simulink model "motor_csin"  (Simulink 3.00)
settings: Solver=ode45  StartTime=0.0  StopTime=2.5  RelTol=1e-6  AbsTol=1e-6
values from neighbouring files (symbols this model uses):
  A = [-Ra Xq ; -Xdp -Ra]    [Gsinc.m]    (also in Cinic.m = -Xs*(Xm+Xr)-Xr*Xm; ptaylor.m = 0; Tdqf.m = [sin(u(3)) cos(u(3)); - cos(u(3)) sin(u(3))]; Tfdq.m = [sin(u(3)) cos(u(3)); - cos(u(3)) sin(u(3))])
  Ac = real(z(1,1))    [ptaylor.m]    (also in workspace_ctes.m = 0.0095)
  As = real(z(1,1))    [ptaylor.m]    (also in workspace_ctes.m = 0.035)
  B = [0 u(3)]'    [Gsinc.m]    (also in Cinic.m = Rs*(Xm+Xr); ptaylor.m = 0; workspace_ctes.m = 0)
  Bc = imag(z(1,1))    [ptaylor.m]    (also in workspace_ctes.m = 0.1279)
  Bs = imag(z(1,1))    [ptaylor.m]    (also in workspace_ctes.m = 0.2438)
  C = Pm*A^2+Pm*B^2-Rs*(Xm+Xr)^2    [Cinic.m]    (also in ptaylor.m = 0; workspace_ctes.m = 0)
  Cc = real(z(2,1))    [ptaylor.m]    (also in workspace_ctes.m = -0.3544)
  Cs = real(z(2,1))    [ptaylor.m]    (also in workspace_ctes.m = -0.678)
  D = 2*Pm*Rs*Rr*A+2*Pm*(Xs*Rr+Rr*Xm)*B-Rr*Xm^2    [Cinic.m]    (also in ptaylor.m = 0; workspace_ctes.m = 0)
  Dc = imag(z(2,1))    [ptaylor.m]    (also in workspace_ctes.m = 0.0093)
  Ds = imag(z(2,1))    [ptaylor.m]    (also in workspace_ctes.m = 0.0644)
  Imv = Imv'    [ptaylor.m]    (also in workspace_ctes.m = [-0.0879 -1.7628 -0.2794 1.4912])
  Imvc = Imvc'    [ptaylor.m]    (also in workspace_ctes.m = [-0.0175 -0.6693 -0.2556 1.8032])
  Imvs = Imvs'    [ptaylor.m]    (also in workspace_ctes.m = [-0.1217 -1.2805 -0.3651 0.9022])
  U3v = U3v'    [ptaylor.m]    (also in workspace_ctes.m = [0.6354 -0.0622 0.4667 -0.0233])
  U3vc = U3vc'    [ptaylor.m]    (also in workspace_ctes.m = [0.2415 -0.0179 0.3544 -0.0093])
  U3vs = U3vs'    [ptaylor.m]    (also in workspace_ctes.m = [0.4605 -0.0661 0.6780 -0.0644])

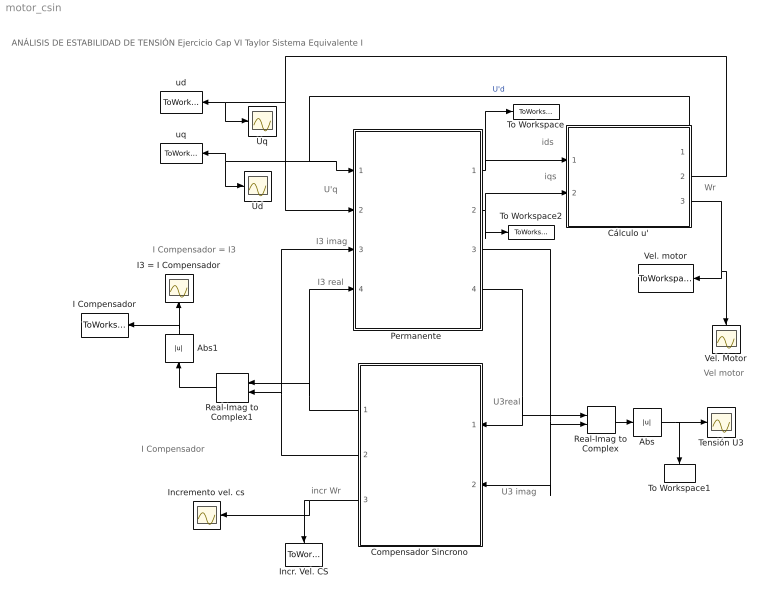
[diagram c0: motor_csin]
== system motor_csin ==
  note: incr Wr
  note: I3 real
  note: I3 imag
  note: U3real
  note: U3 imag
  note: U'q
  note: ids
  note: iqs
  note: Wr
  note: Vel motor
  note: I Compensador
  note: I Compensador = I3
  note: ANÁLISIS DE ESTABILIDAD DE TENSIÓN Ejercicio Cap VI Taylor Sistema Equivalente I
  Abs : Abs
  Abs1 : Abs  Orientation=up
  Compensador Sincrono : Subsystem  Orientation=left  mask{Xd=5.544, Xq=3.26, Xdp=1.14, Ra=0, H=0.5375, Xt=0.34, Emin=-9, Emax=12.43, Tdp=9.564, K=100}
      mask prompts: Xd "Reactancia Síncrona  de Eje d ,  Xd  (p.u.)"; Xq "Reactancia Síncrona  de Eje q,  Xq  (p.u.)"; Xdp "Reactancia Subtransitoria de eje d,  X'd  (p.u.)"; Ra "Resistencia de Estator,  Ra  (p.u.)"; H "Constante de Inercia H (s)"; Xt "Reactancia del transformador,  Xt  (p.u.)"; Emin "Limite Inferior Regulador de Tensión"; Emax "Límite Superior Regulador"; Tdp "Constante de Tiempo del Rotor (s)"; K "Ganancia del Regulador"
  Cálculo u' : Subsystem  mask(Modelo del rotor  del motor){Um=1, Pm=0.6, Am=1, Bm=0, Cm=0, Dm=0, Hm=0.7, Xm=3.2, Xr=0.18, Rr=0.018, Xs=0.1, Rs=0.031}
      mask prompts: Um "Tensión de alimentación (p.u)"; Pm "Potencia en el eje (p.u.)"; Am "Parámetro A modelo de Tcarga"; Bm "Parámetro B modelo de Tcarga"; Cm "Parámetro C modelo de Tcarga"; Dm "Parámetro D modelo de Tcarga"; Hm "Inercia,  H (s)"; Xm "Reactancia de Magnetización,  Xm (p.u.)"; Xr "Reactancia Rotor,  Xr  (p.u.)"; Rr "Resistencia del Rotor,  Rr  (p.u.)"; Xs "Reactancia del estator,  Xs  (p.u.)"; Rs "Resistencia del estator,  Rs  (p.u.)"
  I Compensador : ToWorkspace  VariableName=ICS  SampleTime=-1  SaveFormat=Matrix
  I3 = I Compensador : Scope
  Incr. Vel. CS : ToWorkspace  VariableName=Wmcs  SampleTime=-1  SaveFormat=Matrix
  Incremento vel. cs : Scope
  "Permanente " : Subsystem
  Real-Imag to Complex : RealImagToComplex  Input=RealAndImag  ConstantPart=0
  Real-Imag to Complex1 : RealImagToComplex  Orientation=left  Input=RealAndImag  ConstantPart=0
  Tensión U3 : Scope
  To Workspace : ToWorkspace  VariableName=ids  SampleTime=0  SaveFormat=Matrix
  To Workspace1 : ToWorkspace  VariableName=U3  SampleTime=-1  SaveFormat=Matrix
  To Workspace2 : ToWorkspace  VariableName=iqs  SampleTime=0  SaveFormat=Matrix
  Ud : Scope
  Uq : Scope
  Vel. Motor : Scope
  Vel. motor : ToWorkspace  VariableName=wr  SampleTime=-1  SaveFormat=Matrix
  ud : ToWorkspace  VariableName=uq  SampleTime=-1  SaveFormat=Matrix
  uq : ToWorkspace  VariableName=ud  SampleTime=-1  SaveFormat=Matrix
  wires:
  Compensador Sincrono/2(I3imag) -> "Permanente "/3(I3imag), Real-Imag to Complex1/2
  Compensador Sincrono/1(I3real) -> "Permanente "/4(I3real), Real-Imag to Complex1/1
  "Permanente "/4(U3real) -> Compensador Sincrono/1(U3real), Real-Imag to Complex/1
  "Permanente "/3(U3 imag) -> Compensador Sincrono/2(U3imag), Real-Imag to Complex/2
  Real-Imag to Complex/1 -> Abs/1
  Abs/1 -> Tensión U3/1, To Workspace1/1
  Cálculo u'/2(u'q) -> "Permanente "/2(u'q), ud/1, Uq/1
  Cálculo u'/1(u'd) -> "Permanente "/1(u'd), uq/1, Ud/1  "U'd"
  Compensador Sincrono/3(Inc Wr) -> Incr. Vel. CS/1, Incremento vel. cs/1
  Cálculo u'/3(wr) -> Vel. motor/1, Vel. Motor/1
  "Permanente "/1(ids) -> Cálculo u'/1(ids), To Workspace/1
  "Permanente "/2(iqs) -> Cálculo u'/2(iqs), To Workspace2/1
  Real-Imag to Complex1/1 -> Abs1/1
  Abs1/1 -> I3 = I Compensador/1, I Compensador/1

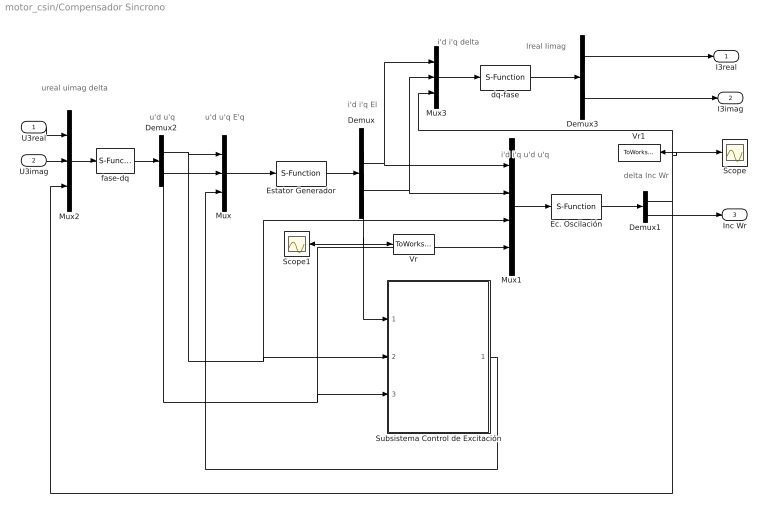
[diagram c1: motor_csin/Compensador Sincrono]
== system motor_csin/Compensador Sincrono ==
  note: u'd u'q E'q
  note: i'd i'q El
  note: i'd i'q u'd u'q
  note: delta Inc Wr
  note: ureal uimag delta
  note: u'd u'q
  note: i'd i'q delta
  note: Ireal Iimag
  U3real : Inport  Port=1  PortWidth=-1  SampleTime=-1  DataType=auto
  U3imag : Inport  Port=2  PortWidth=-1  SampleTime=-1  DataType=auto
  Demux : Demux  Outputs=3
  Demux1 : Demux  Outputs=2
  Demux2 : Demux  Outputs=2
  Demux3 : Demux  Outputs=2
  Ec. Oscilación : S-Function  FunctionName=geosc  Parameters=H  PortCounts=[]  SFunctionModules=''
  Estator Generador : S-Function  FunctionName=gsinc  Parameters=Ra, Xd, Xq, Xdp, Xt  PortCounts=[]  SFunctionModules=''
  Mux : Mux  Inputs=3
  Mux1 : Mux  Inputs=4
  Mux2 : Mux  Inputs=3
  Mux3 : Mux  Inputs=3
  Scope : Scope
  Scope1 : Scope
  Subsistema Control de Excitación : Subsystem  mask{Tdp=Tdp, Emax=Emax, Emin=Emin, K=K}
      mask prompts: Tdp "Cte. Tiempo Rotor"; K "Ganancia Regulador"
  Vr : ToWorkspace  VariableName=El  SampleTime=-1  SaveFormat=Matrix
  Vr1 : ToWorkspace  VariableName=delta  SampleTime=-1  SaveFormat=Matrix
  dq-fase : S-Function  FunctionName=Tdqf  PortCounts=[]  SFunctionModules=''
  fase-dq : S-Function  FunctionName=Tfdq  PortCounts=[]  SFunctionModules=''
  I3real : Outport  Port=1
  I3imag : Outport  Port=2
  Inc Wr : Outport  Port=3
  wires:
  Mux3/1 -> dq-fase/1
  dq-fase/1 -> Demux3/1
  Demux3/1 -> I3real/1
  Demux3/2 -> I3imag/1
  Mux1/1 -> Ec. Oscilación/1
  Demux/1 -> Mux1/1, Mux3/1
  Demux/2 -> Mux1/2, Mux3/2
  Estator Generador/1 -> Demux/1
  Mux2/1 -> fase-dq/1
  U3real/1 -> Mux2/1
  U3imag/1 -> Mux2/2
  fase-dq/1 -> Demux2/1
  Demux2/1 -> Mux/1, Subsistema Control de Excitación/2(u'd), Mux1/3
  Demux2/2 -> Mux/2, Subsistema Control de Excitación/3(u'q), Mux1/4
  Mux/1 -> Estator Generador/1
  Subsistema Control de Excitación/1(E'q) -> Mux/3
  Ec. Oscilación/1 -> Demux1/1
  Demux1/2 -> Inc Wr/1
  Demux1/1 -> Mux2/3, Mux3/3, Scope/1, Vr1/1
  Demux/3 -> Subsistema Control de Excitación/1(E l), Scope1/1, Vr/1

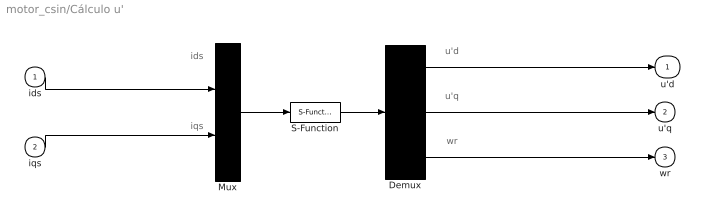
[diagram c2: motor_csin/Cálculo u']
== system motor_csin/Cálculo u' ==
  note: wr
  note: u'q
  note: u'd
  note: iqs
  note: ids
  ids : Inport  Port=1  PortWidth=-1  SampleTime=-1  DataType=auto
  iqs : Inport  Port=2  PortWidth=-1  SampleTime=-1  DataType=auto
  Demux : Demux  Outputs=3
  Mux : Mux  Inputs=2
  S-Function : S-Function  FunctionName=rotorind  Parameters=Rs, Xs, Rr, Xr, Xm, Hm, Am, Bm, Cm, Dm, Pm, Um  PortCounts=[]  SFunctionModules=''
  u'd : Outport  Port=1
  u'q : Outport  Port=2
  wr : Outport  Port=3
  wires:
  ids/1 -> Mux/1
  iqs/1 -> Mux/2
  S-Function/1 -> Demux/1
  Mux/1 -> S-Function/1
  Demux/1 -> u'd/1
  Demux/2 -> u'q/1
  Demux/3 -> wr/1

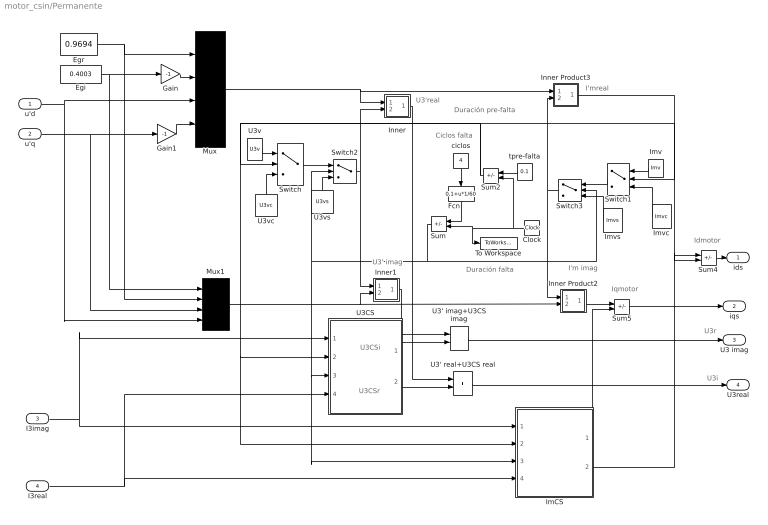
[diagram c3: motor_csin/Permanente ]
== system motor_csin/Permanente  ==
  note: U3'real
  note: U3' imag
  note: I'mreal
  note: I'm imag
  note: Idmotor
  note: U3CSi
  note: U3CSr
  note: Iqmotor
  note: U3r
  note: U3i
  note: Ciclos falta
  note: Duración pre-falta
  note: Duración falta
  u'd : Inport  Port=1  PortWidth=-1  SampleTime=-1  DataType=auto
  u'q : Inport  Port=2  PortWidth=-1  SampleTime=-1  DataType=auto
  I3imag : Inport  Port=3  PortWidth=-1  SampleTime=-1  DataType=auto
  I3real : Inport  Port=4  PortWidth=-1  SampleTime=-1  DataType=auto
  Clock : Clock
  Egi : Constant  Value=0.4003
  Egr : Constant  Value=0.9694
  Fcn : Fcn  Orientation=down  Expr=0.1+u*1/60
  Gain : Gain  Gain=-1  SaturateOnIntegerOverflow=on
  Gain1 : Gain  Gain=-1  SaturateOnIntegerOverflow=on
  ImCS : Subsystem
  Imv : Constant  Orientation=left  Value=Imv
  Imvc : Constant  Orientation=left  Value=Imvc
  Imvs : Constant  Orientation=left  Value=Imvs
  Inner : Subsystem
  Inner Product2 : Subsystem
  Inner Product3 : Subsystem
  Inner1 : Subsystem
  Mux : Mux  Inputs=4
  Mux1 : Mux  Inputs=4
  Sum : Sum  Orientation=left  Inputs=+-  SaturateOnIntegerOverflow=on
  Sum2 : Sum  Orientation=left  Inputs=+-  SaturateOnIntegerOverflow=on
  Sum4 : Sum  Inputs=+-  SaturateOnIntegerOverflow=on
  Sum5 : Sum  Inputs=+-  SaturateOnIntegerOverflow=on
  Switch : Switch  Threshold=0
  Switch1 : Switch  Orientation=left  Threshold=0
  Switch2 : Switch  Threshold=0
  Switch3 : Switch  Orientation=left  Threshold=0
  To Workspace : ToWorkspace  VariableName=t  SampleTime=0  SaveFormat=Matrix
  U3' imag+U3CS imag : Sum  Inputs=++  SaturateOnIntegerOverflow=on
  U3' real+U3CS real : Sum  Inputs=++  SaturateOnIntegerOverflow=on
  U3CS : Subsystem
  U3v : Constant  Value=U3v
  U3vc : Constant  Orientation=up  Value=U3vc
  U3vs : Constant  Orientation=up  Value=U3vs
  ciclos : Constant  Orientation=down  Value=4
  tpre-falta : Constant  Orientation=left  Value=0.1
  ids : Outport  Port=1
  iqs : Outport  Port=2
  U3 imag : Outport  Port=3
  U3real : Outport  Port=4
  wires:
  U3vc/1 -> Switch/3
  U3v/1 -> Switch/1
  Switch/1 -> Switch2/1
  U3vs/1 -> Switch2/3
  Sum/1 -> Switch3/2, Switch2/2, ImCS/3(T falta), U3CS/3(T falta)
  Imvc/1 -> Switch1/3
  Imv/1 -> Switch1/1
  Fcn/1 -> Sum/1
  tpre-falta/1 -> Sum2/1
  Sum2/1 -> Switch1/2, Switch/2, ImCS/2(T pre-falta), U3CS/2(T Pre-falta)
  Switch1/1 -> Switch3/1
  Imvs/1 -> Switch3/3
  ciclos/1 -> Fcn/1
  Inner Product3/1(out_1) -> Sum4/1
  Egr/1 -> Mux/1, Mux1/2
  Mux1/1 -> Inner Product2/2(in_2), Inner1/2(in_2)
  Inner/1(out_1) -> U3' real+U3CS real/1
  U3CS/2(U3CS real) -> U3' real+U3CS real/2
  U3CS/1(U3CS imag.) -> U3' imag+U3CS imag/2
  Inner1/1(out_1) -> U3' imag+U3CS imag/1
  Inner Product2/1(out_1) -> Sum5/1
  I3real/1 -> ImCS/4(I3 real), U3CS/4(I3 real)
  I3imag/1 -> ImCS/1(I3 imag.), U3CS/1(I3 imag.)
  Sum4/1 -> ids/1
  Sum5/1 -> iqs/1
  U3' imag+U3CS imag/1 -> U3 imag/1
  U3' real+U3CS real/1 -> U3real/1
  Gain1/1 -> Mux/4
  u'q/1 -> Gain1/1, Mux1/3
  u'd/1 -> Mux/3, Mux1/4
  Gain/1 -> Mux/2
  Egi/1 -> Gain/1, Mux1/1
  Switch3/1 -> Inner Product2/1(in_1), Inner Product3/2(in_2)
  Switch2/1 -> Inner1/1(in_1), Inner/2(in_2)
  Mux/1 -> Inner Product3/1(in_1), Inner/1(in_1)
  Clock/1 -> Sum/2, To Workspace/1, Sum2/2
  ImCS/2(ImCS real) -> Sum4/2
  ImCS/1(ImCS imag) -> Sum5/2

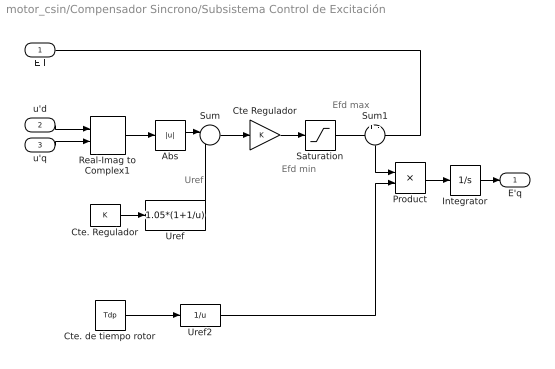
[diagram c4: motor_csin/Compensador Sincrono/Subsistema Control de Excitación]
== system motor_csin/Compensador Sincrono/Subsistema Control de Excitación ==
  note: Uref
  note: Efd max
  note: Efd min
  E l : Inport  Port=1  PortWidth=-1  SampleTime=-1  DataType=auto
  u'd : Inport  Port=2  PortWidth=-1  SampleTime=-1  DataType=auto
  u'q : Inport  Port=3  PortWidth=-1  SampleTime=-1  DataType=auto
  Abs : Abs
  Cte Regulador : Gain  Gain=K  SaturateOnIntegerOverflow=on
  Cte. Regulador : Constant  Value=K
  Cte. de tiempo rotor : Constant  Value=Tdp
  Integrator : Integrator  ExternalReset=none  InitialConditionSource=internal  InitialCondition=1.05  LimitOutput=off  UpperSaturationLimit=inf  LowerSaturationLimit=-inf  ShowSaturationPort=off  ShowStatePort=off  AbsoluteTolerance=auto
  Product : Product  Inputs=2  SaturateOnIntegerOverflow=on
  Real-Imag to Complex1 : RealImagToComplex  Input=RealAndImag  ConstantPart=0
  Saturation : Saturate  UpperLimit=Emax  LowerLimit=Emin
  Sum : Sum  Inputs=|-+  SaturateOnIntegerOverflow=on
  Sum1 : Sum  Orientation=down  Inputs=+-  SaturateOnIntegerOverflow=on
  Uref : Fcn  Expr=1.05*(1+1/u)
  Uref2 : Fcn  Expr=1/u
  E'q : Outport  Port=1
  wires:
  Sum/1 -> Cte Regulador/1
  Cte Regulador/1 -> Saturation/1
  Abs/1 -> Sum/1
  Cte. Regulador/1 -> Uref/1
  Uref/1 -> Sum/2
  Saturation/1 -> Sum1/1
  E l/1 -> Sum1/2
  Product/1 -> Integrator/1
  Integrator/1 -> E'q/1
  Sum1/1 -> Product/1
  Cte. de tiempo rotor/1 -> Uref2/1
  Uref2/1 -> Product/2
  Real-Imag to Complex1/1 -> Abs/1
  u'd/1 -> Real-Imag to Complex1/1
  u'q/1 -> Real-Imag to Complex1/2

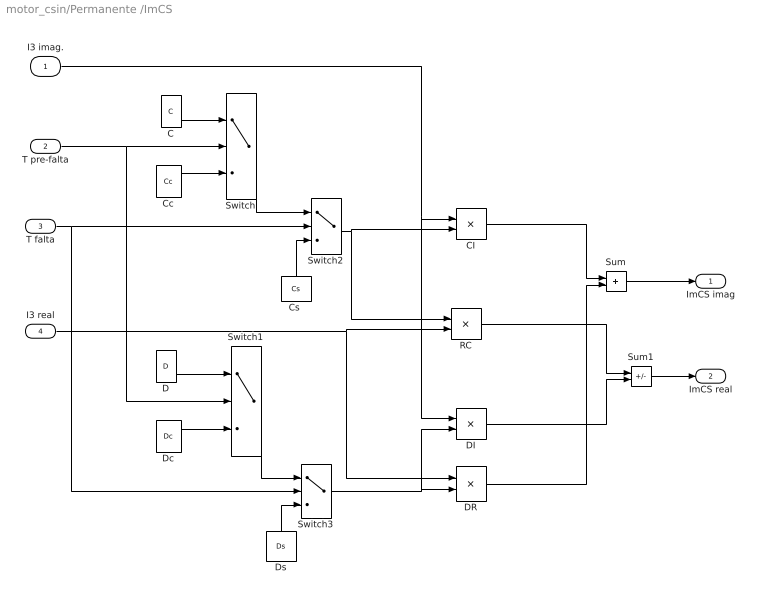
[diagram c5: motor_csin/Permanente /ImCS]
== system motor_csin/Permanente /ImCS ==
  I3 imag. : Inport  Port=1  PortWidth=-1  SampleTime=-1  DataType=auto
  T pre-falta : Inport  Port=2  PortWidth=-1  SampleTime=-1  DataType=auto
  T falta : Inport  Port=3  PortWidth=-1  SampleTime=-1  DataType=auto
  I3 real : Inport  Port=4  PortWidth=-1  SampleTime=-1  DataType=auto
  C : Constant  Value=C
  CI : Product  Inputs=2  SaturateOnIntegerOverflow=on
  Cc : Constant  Value=Cc
  "Cs " : Constant  Orientation=up  Value=Cs
  D : Constant  Value=D
  DI : Product  Inputs=2  SaturateOnIntegerOverflow=on
  DR : Product  Inputs=2  SaturateOnIntegerOverflow=on
  Dc : Constant  Value=Dc
  Ds : Constant  Orientation=up  Value=Ds
  RC : Product  Inputs=2  SaturateOnIntegerOverflow=on
  Sum : Sum  Inputs=++  SaturateOnIntegerOverflow=on
  Sum1 : Sum  Inputs=+-  SaturateOnIntegerOverflow=on
  Switch{,1..3} (4 alike) : Switch  Threshold=0
  ImCS imag : Outport  Port=1
  ImCS real : Outport  Port=2
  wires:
  Ds/1 -> Switch3/3
  Cc/1 -> Switch/3
  C/1 -> Switch/1
  T pre-falta/1 -> Switch/2, Switch1/2
  T falta/1 -> Switch2/2, Switch3/2
  Switch1/1 -> Switch3/1
  Dc/1 -> Switch1/3
  D/1 -> Switch1/1
  Switch/1 -> Switch2/1
  "Cs "/1 -> Switch2/3
  I3 imag./1 -> CI/1, DI/1
  Switch3/1 -> DR/2, DI/2
  Sum1/1 -> ImCS real/1
  I3 real/1 -> DR/1, RC/2
  Switch2/1 -> CI/2, RC/1
  DI/1 -> Sum1/2
  DR/1 -> Sum/2
  Sum/1 -> ImCS imag/1
  CI/1 -> Sum/1
  RC/1 -> Sum1/1

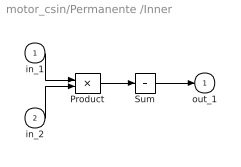
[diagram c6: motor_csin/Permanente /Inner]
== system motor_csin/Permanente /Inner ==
  in_1 : Inport  Port=1  PortWidth=-1  SampleTime=-1  DataType=auto
  in_2 : Inport  Port=2  PortWidth=-1  SampleTime=-1  DataType=auto
  Product : Product  Inputs=2  SaturateOnIntegerOverflow=on
  Sum : Sum  Inputs=+  SaturateOnIntegerOverflow=on
  out_1 : Outport  Port=1
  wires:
  in_2/1 -> Product/2
  in_1/1 -> Product/1
  Product/1 -> Sum/1
  Sum/1 -> out_1/1

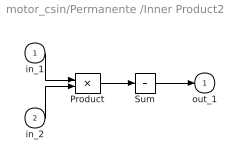
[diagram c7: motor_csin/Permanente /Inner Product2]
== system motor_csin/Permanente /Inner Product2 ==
  in_1 : Inport  Port=1  PortWidth=-1  SampleTime=-1  DataType=auto
  in_2 : Inport  Port=2  PortWidth=-1  SampleTime=-1  DataType=auto
  Product : Product  Inputs=2  SaturateOnIntegerOverflow=on
  Sum : Sum  Inputs=+  SaturateOnIntegerOverflow=on
  out_1 : Outport  Port=1
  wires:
  in_2/1 -> Product/2
  in_1/1 -> Product/1
  Product/1 -> Sum/1
  Sum/1 -> out_1/1

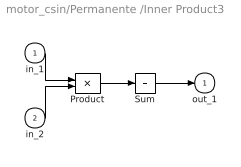
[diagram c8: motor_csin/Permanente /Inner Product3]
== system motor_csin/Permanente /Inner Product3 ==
  in_1 : Inport  Port=1  PortWidth=-1  SampleTime=-1  DataType=auto
  in_2 : Inport  Port=2  PortWidth=-1  SampleTime=-1  DataType=auto
  Product : Product  Inputs=2  SaturateOnIntegerOverflow=on
  Sum : Sum  Inputs=+  SaturateOnIntegerOverflow=on
  out_1 : Outport  Port=1
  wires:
  in_2/1 -> Product/2
  in_1/1 -> Product/1
  Product/1 -> Sum/1
  Sum/1 -> out_1/1

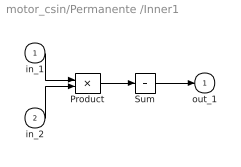
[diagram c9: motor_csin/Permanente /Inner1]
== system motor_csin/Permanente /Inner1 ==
  in_1 : Inport  Port=1  PortWidth=-1  SampleTime=-1  DataType=auto
  in_2 : Inport  Port=2  PortWidth=-1  SampleTime=-1  DataType=auto
  Product : Product  Inputs=2  SaturateOnIntegerOverflow=on
  Sum : Sum  Inputs=+  SaturateOnIntegerOverflow=on
  out_1 : Outport  Port=1
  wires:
  in_2/1 -> Product/2
  in_1/1 -> Product/1
  Product/1 -> Sum/1
  Sum/1 -> out_1/1

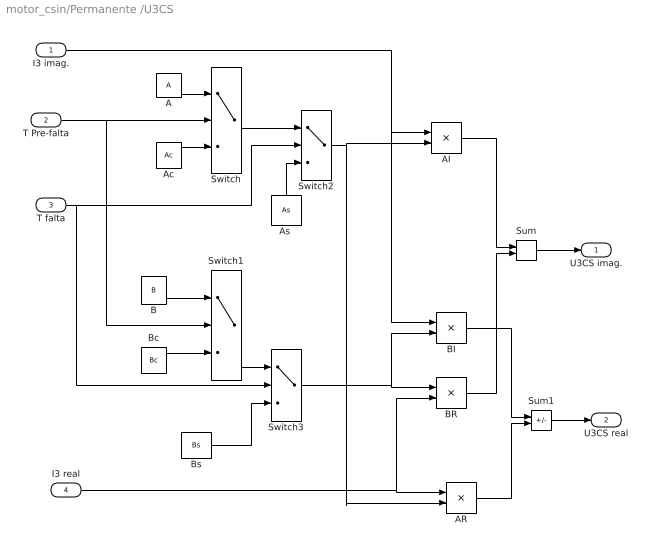
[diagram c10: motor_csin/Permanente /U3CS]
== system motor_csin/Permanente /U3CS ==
  I3 imag. : Inport  Port=1  PortWidth=-1  SampleTime=-1  DataType=auto
  T Pre-falta : Inport  Port=2  PortWidth=-1  SampleTime=-1  DataType=auto
  T falta : Inport  Port=3  PortWidth=-1  SampleTime=-1  DataType=auto
  I3 real : Inport  Port=4  PortWidth=-1  SampleTime=-1  DataType=auto
  A : Constant  Value=A
  AI : Product  Inputs=2  SaturateOnIntegerOverflow=on
  AR : Product  Inputs=2  SaturateOnIntegerOverflow=on
  Ac : Constant  Value=Ac
  "As " : Constant  Orientation=up  Value=As
  B : Constant  Value=B
  BI : Product  Inputs=2  SaturateOnIntegerOverflow=on
  BR : Product  Inputs=2  SaturateOnIntegerOverflow=on
  Bc : Constant  Value=Bc
  Bs : Constant  Value=Bs
  Sum : Sum  Inputs=++  SaturateOnIntegerOverflow=on
  Sum1 : Sum  Inputs=-+  SaturateOnIntegerOverflow=on
  Switch{,1..3} (4 alike) : Switch  Threshold=0
  U3CS imag. : Outport  Port=1
  U3CS real : Outport  Port=2
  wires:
  Switch/1 -> Switch2/1
  "As "/1 -> Switch2/3
  Ac/1 -> Switch/3
  A/1 -> Switch/1
  T Pre-falta/1 -> Switch/2, Switch1/2
  T falta/1 -> Switch2/2, Switch3/2
  AI/1 -> Sum/1
  BR/1 -> Sum/2
  I3 imag./1 -> AI/1, BI/1
  Switch2/1 -> AI/2, AR/2
  BI/1 -> Sum1/1
  Sum/1 -> U3CS imag./1
  Sum1/1 -> U3CS real/1
  Switch1/1 -> Switch3/1
  Bs/1 -> Switch3/3
  Bc/1 -> Switch1/3
  B/1 -> Switch1/1
  I3 real/1 -> AR/1, BR/2
  Switch3/1 -> BR/1, BI/2
  AR/1 -> Sum1/2
